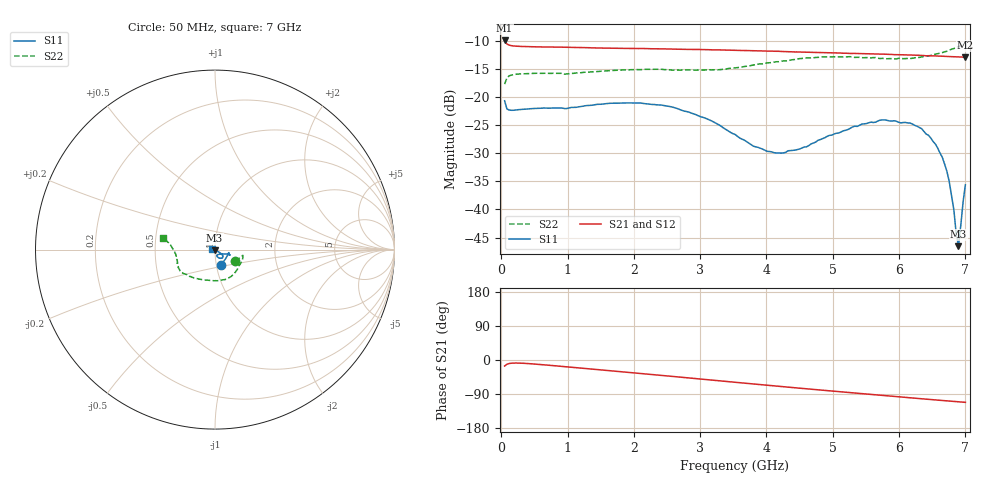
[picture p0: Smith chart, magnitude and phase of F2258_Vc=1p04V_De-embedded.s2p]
! Integrated Device Technology
! Corporate Headquarters
! 6024 Silver Creek Valley Road
! San Jose, CA 95138  USA
! Phone:  1-408-284-8200
! Toll Free:  1-800-223-1366
! Webpage:  http://www.idt.com/
! Timing and RF Division
! 515 Groton Road, Suite 102
! Westford, MA 01886-6024
! Device:  F2258
! Description: Voltage Variable RF Attenuator
! Frequency:  50.0 -  6000.00 MHz
! Package:  3x3 mm Thin QFN Plastic Package: 16 pin
! Ports:  2 RF, 2 DC
!  Pin  1  = NC
!  Pin  2  = NC
!  Pin  3  = RF2  = Port 2
!  Pin  4  = GND
!  Pin  5  = Vdd
!  Pin  6  = NC
!  Pin  7  = VCTRL
!  Pin  8  = NC
!  Pin  9  = GND
!  Pin 10  = RF1  = Port 1
!  Pin 11  = NC
!  Pin 12  = NC
!  Pin 13  = NC
!  Pin 14  = NC
!  Pin 15  = NC
!  Pin 16  = NC
! Vcntrl:  1.040 Volts
! Vdd:  +3.300 Volts
! Current:  1.159 mA
! Data:  The device was measured on a the F2258 evaluation board which has
!  individual transmission lines to the RF pins.  Data was collected
!  using a calibrated network analyzer.  The evaluation board was
!  de-embedded using a TRL calibration technique.
!  The reference plane is the edge of the package pin.
! Misc:  SN 10
!  Action Tracker AT0285
! Date Measured:  2014-12-10
! Date:  2016-01-13  MJV
! Note:
!  Integrated Device Technology supplies this data as a sample of measured
!  data at the package pin for this product.  Your particular data for this
!  product may vary.
!  Data was taken at 25 degrees C.
!  Integrated Device Technology reserves the right to change this data at anytime.
!Freq_(GHz)  S11M_(dB)  S11P_(deg)  S21M_(dB)  S21P_(deg)  S12M_(dB)  S12P_(deg)  S22M_(dB)  S22P_(deg)
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# GHz S dB R 50
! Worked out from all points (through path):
!   201 points, 50 MHz to 7 GHz, reference 50 ohm
!   highest |S21| = -9.95 dB at 50 MHz (marker M1); lowest = -12.9 dB at 7 GHz (marker M2)
!   group delay of S21, straight-line fit = 43.4 ps
!   lowest |S11| = -46.5 dB at 6.896 GHz (marker M3), VSWR 1.01, Z = 49.7 - j0.393 ohm
!   |S11| at or under -10 dB: start of sweep to end of sweep
!   |S22| runs from -17.7 to -10.5 dB; largest |S21 - S12| = 0.001
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0.05  -20.68 -69.7  -9.95 -15.9  -9.94 -15.9  -17.71 -29.9
0.08475  -22.14 -41.9  -10.57 -11.2  -10.56 -11.2  -16.61 -16.5
0.15425  -22.37 -22.5  -10.88 -8.4  -10.86 -8.4  -16.10 -12.3
1.2315  -21.65 -18.6  -11.23 -21.9  -11.21 -21.9  -15.63 -40.3
2.37825  -21.43 -19.3  -11.45 -40.0  -11.44 -40.0  -15.08 -70.8
3.07325  -23.75 -22.7  -11.58 -51.3  -11.58 -51.3  -15.20 -94.2
3.525  -26.66 -31.7  -11.69 -58.7  -11.70 -58.7  -14.83 -112.5
3.803  -28.75 -45.1  -11.76 -63.3  -11.77 -63.2  -14.31 -123.1
4.1505  -29.98 -61.4  -11.87 -68.8  -11.88 -68.8  -13.73 -133.5
4.7065  -28.21 -73.1  -12.07 -77.5  -12.07 -77.5  -13.03 -145.9
5.43625  -24.83 -58.5  -12.30 -88.6  -12.28 -88.7  -13.01 -157.1
5.85325  -24.26 -46.6  -12.42 -94.9  -12.42 -95.0  -13.18 -165.3
6.166  -24.65 -40.8  -12.52 -99.7  -12.54 -99.7  -13.17 -172.6
6.33975  -25.64 -36.5  -12.61 -102.3  -12.63 -102.3  -12.89 -177.4
6.583  -29.11 -32.8  -12.73 -105.9  -12.73 -105.8  -12.32 176.3
6.6525  -30.74 -31.6  -12.75 -106.9  -12.75 -106.9  -12.11 174.4
6.75675  -35.08 -36.3  -12.81 -108.4  -12.83 -108.4  -11.68 171.6
6.82625  -40.11 -48.5  -12.83 -109.3  -12.85 -109.3  -11.39 170.5
6.861  -44.27 -68.4  -12.85 -109.9  -12.86 -109.8  -11.23 169.7
6.89575  -46.54 -123.0  -12.88 -110.3  -12.89 -110.3  -11.03 169.0
6.96525  -38.69 -170.5  -12.91 -111.3  -12.91 -111.3  -10.75 167.7
7  -35.62 176.3  -12.92 -111.7  -12.92 -111.8  -10.54 166.9
